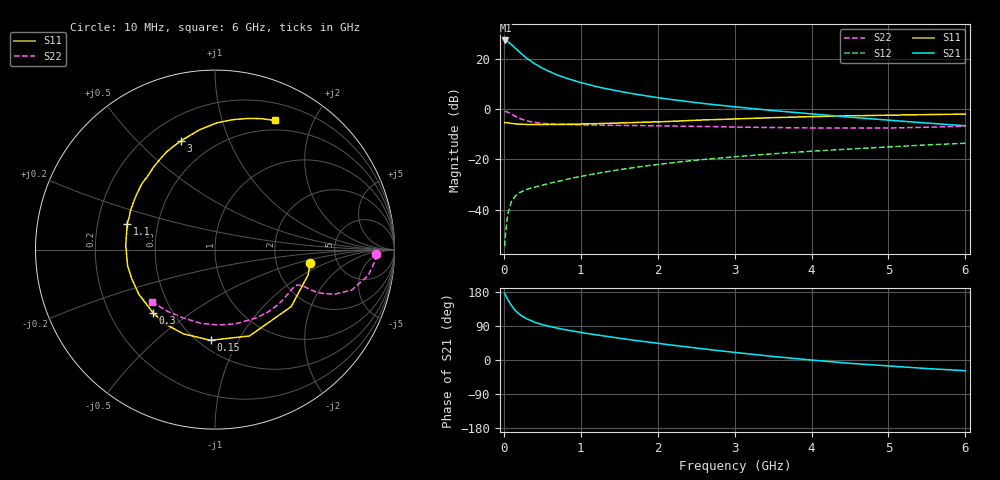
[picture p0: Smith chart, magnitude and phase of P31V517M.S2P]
! SIEMENS Small Signal Semiconductors
! BFP181
! Si NPN RF Bipolar Junction Transistor in SOT143
! VCE = 1.5 V  IC = 17 mA
! Common Emitter S-Parameters:  March  1996
# GHz  S  MA  R  50
!  f  S11  S21  S12  S22
! GHz  MAG  ANG  MAG  ANG  MAG  ANG  MAG  ANG
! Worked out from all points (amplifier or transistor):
!   36 points, 10 MHz to 6 GHz, reference 50 ohm
!   highest |S21| = 27.2 dB at 20 MHz (marker M1)
!   |S21| within 3 dB of that: start of sweep to 147.3 MHz
!   unconditionally stable (mu >= 1): start of sweep to 21.61 MHz; 350 MHz to end of sweep
!   at 250 MHz: K = 0.80, MSG = 26.9 dB, |S12| = -32.6 dB
!   at 1.4 GHz: K = 1.81, MAG = 10.9 dB, |S12| = -24.6 dB
!   at 6 GHz: K = 1.43, MAG = -0.4 dB, |S12| = -13.6 dB
!   S11 on the Smith chart (normalised r, x): 10 MHz: 3.16, -0.65; 150 MHz: 0.57, -0.77; 300 MHz: 0.39, -0.36; 1.1 GHz: 0.33, +0.13; 3 GHz: 0.33, +0.68; 6 GHz: 0.39, +1.49
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0.01  0.5363 -7.9  22.88 175.9  0.0019 78.3  0.8978 -1.7
0.02  0.5372 -15.4  22.9 172.1  0.003 77.7  0.8953 -3.8
0.05  0.5302 -36.8  21.88 160.1  0.0082 76.8  0.8658 -9.6
0.1  0.5181 -68.2  18.92 143.6  0.0146 62.0  0.7941 -16.5
0.15  0.5059 -92.8  16.07 130.7  0.0188 54.8  0.7147 -20.3
0.2  0.5012 -110.6  13.66 121.2  0.022 50.8  0.6559 -22.0
0.25  0.4989 -123.9  11.64 114.1  0.0235 47.6  0.6128 -22.7
0.3  0.4931 -134.6  10.11 108.6  0.0256 46.6  0.5816 -22.8
0.4  0.4919 -149.7  7.95 99.9  0.0283 46.6  0.542 -22.5
0.5  0.4914 -160.8  6.466 93.5  0.0308 47.0  0.5197 -22.7
0.6  0.4952 -169.5  5.48 88.4  0.0339 48.9  0.5064 -22.9
0.7  0.4933 -176.1  4.695 83.8  0.0365 50.2  0.4973 -23.5
0.8  0.4968 177.9  4.158 79.8  0.0394 51.0  0.4916 -24.4
1  0.5024 168.1  3.345 72.8  0.0458 53.2  0.4837 -26.5
1.1  0.5101 163.5  3.062 69.4  0.0493 53.4  0.4809 -27.8
1.5  0.5276 148.7  2.249 57.4  0.0624 54.5  0.4732 -33.7
2.2  0.5719 127.1  1.527 38.9  0.0861 52.2  0.4588 -46.3
3  0.6353 107.3  1.105 20.1  0.1128 47.0  0.4381 -62.8
3.5  0.6734 97.3  0.931 9.3  0.1293 43.6  0.4289 -74.6
4.5  0.7313 82.0  0.69 -8.8  0.1608 35.2  0.4183 -101.0
5.5  0.774 70.5  0.526 -22.6  0.1941 26.9  0.4343 -127.7
6  0.793 65.2  0.465 -28.2  0.2093 22.1  0.4549 -140.1
